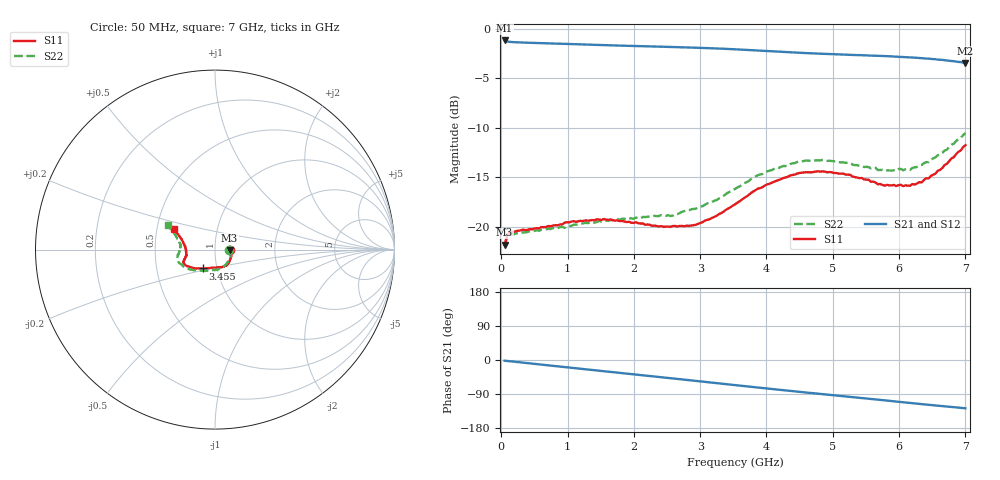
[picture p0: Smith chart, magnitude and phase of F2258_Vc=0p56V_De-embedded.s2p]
! Integrated Device Technology
! Corporate Headquarters
! 6024 Silver Creek Valley Road
! San Jose, CA 95138  USA
! Phone:  1-408-284-8200
! Toll Free:  1-800-223-1366
! Webpage:  http://www.idt.com/
! Timing and RF Division
! 515 Groton Road, Suite 102
! Westford, MA 01886-6024
! Device:  F2258
! Description: Voltage Variable RF Attenuator
! Frequency:  50.0 -  6000.00 MHz
! Package:  3x3 mm Thin QFN Plastic Package: 16 pin
! Ports:  2 RF, 2 DC
!  Pin  1  = NC
!  Pin  2  = NC
!  Pin  3  = RF2  = Port 2
!  Pin  4  = GND
!  Pin  5  = Vdd
!  Pin  6  = NC
!  Pin  7  = VCTRL
!  Pin  8  = NC
!  Pin  9  = GND
!  Pin 10  = RF1  = Port 1
!  Pin 11  = NC
!  Pin 12  = NC
!  Pin 13  = NC
!  Pin 14  = NC
!  Pin 15  = NC
!  Pin 16  = NC
! Vcntrl:  0.560 Volts
! Vdd:  +3.300 Volts
! Current:  1.101 mA
! Data:  The device was measured on a the F2258 evaluation board which has
!  individual transmission lines to the RF pins.  Data was collected
!  using a calibrated network analyzer.  The evaluation board was
!  de-embedded using a TRL calibration technique.
!  The reference plane is the edge of the package pin.
! Misc:  SN 10
!  Action Tracker AT0285
! Date Measured:  2014-12-10
! Date:  2016-01-13  MJV
! Note:
!  Integrated Device Technology supplies this data as a sample of measured
!  data at the package pin for this product.  Your particular data for this
!  product may vary.
!  Data was taken at 25 degrees C.
!  Integrated Device Technology reserves the right to change this data at anytime.
!Freq_(GHz)  S11M_(dB)  S11P_(deg)  S21M_(dB)  S21P_(deg)  S12M_(dB)  S12P_(deg)  S22M_(dB)  S22P_(deg)
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# GHz S dB R 50
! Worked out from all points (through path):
!   201 points, 50 MHz to 7 GHz, reference 50 ohm
!   highest |S21| = -1.19 dB at 50 MHz (marker M1); lowest = -3.5 dB at 7 GHz (marker M2)
!   group delay of S21, straight-line fit = 50.5 ps
!   lowest |S11| = -21.8 dB at 50 MHz (marker M3), VSWR 1.18, Z = 58.8 - j0.476 ohm
!   |S11| at or under -10 dB: start of sweep to end of sweep
!   |S22| runs from -22.0 to -10.6 dB; largest |S21 - S12| = 0.00068
!   S11 on the Smith chart (normalised r, x): 50 MHz: 1.18, -0.01; 3.455 GHz: 0.85, -0.18; 7 GHz: 0.61, +0.15
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0.05  -21.83 -2.8  -1.19 -2.0  -1.19 -2.0  -21.98 -3.0
0.08475  -20.95 -4.6  -1.28 -2.5  -1.28 -2.5  -21.13 -4.7
0.15425  -20.53 -7.1  -1.35 -3.7  -1.35 -3.7  -20.79 -8.2
0.71025  -19.95 -29.7  -1.48 -14.1  -1.48 -14.1  -20.21 -33.9
1.2315  -19.44 -48.8  -1.59 -23.9  -1.59 -23.9  -19.69 -56.9
1.6485  -19.27 -59.5  -1.68 -31.5  -1.68 -31.5  -19.35 -70.0
2.37825  -19.99 -77.8  -1.81 -44.8  -1.81 -44.8  -18.93 -88.8
2.552  -20.03 -83.4  -1.84 -48.0  -1.84 -48.0  -18.94 -94.1
2.93425  -19.82 -99.5  -1.92 -55.1  -1.92 -55.1  -18.20 -107.8
3.247  -18.92 -113.5  -2.00 -61.0  -2.00 -61.0  -17.32 -120.2
3.4555  -18.05 -123.2  -2.06 -64.9  -2.06 -64.9  -16.44 -128.1
3.525  -17.76 -125.7  -2.08 -66.2  -2.09 -66.2  -16.20 -131.2
4.0115  -15.74 -141.9  -2.26 -75.3  -2.26 -75.3  -14.41 -147.5
4.46325  -14.63 -151.6  -2.43 -83.4  -2.42 -83.4  -13.47 -159.1
4.7065  -14.49 -155.0  -2.49 -87.7  -2.50 -87.7  -13.36 -163.5
5.2625  -14.77 -161.5  -2.65 -97.4  -2.65 -97.4  -13.56 -171.9
5.6795  -15.73 -167.4  -2.73 -104.6  -2.74 -104.6  -14.29 -177.7
5.85325  -15.84 -171.6  -2.79 -107.7  -2.79 -107.7  -14.33 177.6
6.166  -15.87 -179.7  -2.89 -113.3  -2.90 -113.3  -14.26 171.3
6.33975  -15.54 173.3  -2.98 -116.4  -2.98 -116.4  -13.78 166.8
6.6525  -14.08 162.3  -3.15 -121.9  -3.16 -121.9  -12.55 159.9
7  -11.77 152.9  -3.45 -127.4  -3.46 -127.4  -10.56 152.4
